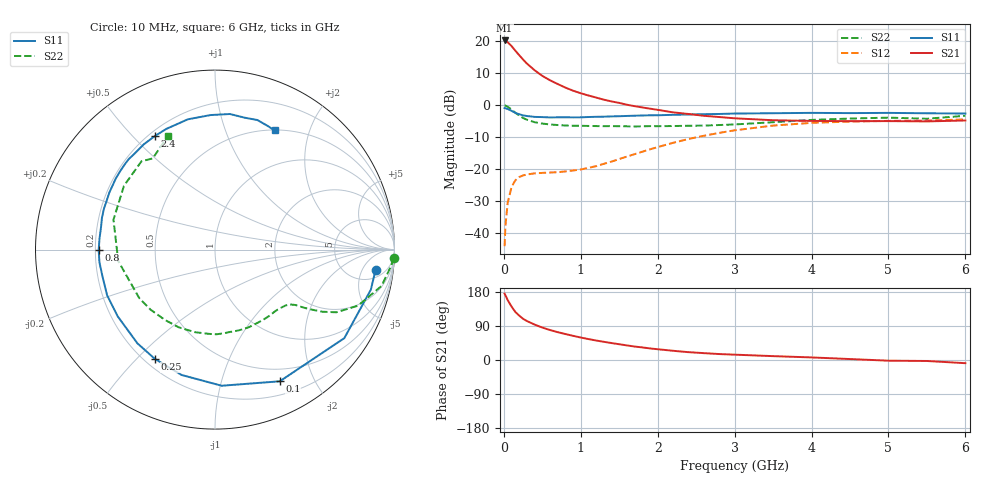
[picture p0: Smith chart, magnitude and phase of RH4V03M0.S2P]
! SIEMENS Small Signal Semiconductors
! BFR106
! Si NPN RF Bipolar Junction Transistor in SOT23
! VCE = 4 V  IC = 3 mA
! Common Emitter S-Parameters:  August  1996
# GHz  S  MA  R  50
!  f  S11  S21  S12  S22
! GHz  MAG  ANG  MAG  ANG  MAG  ANG  MAG  ANG
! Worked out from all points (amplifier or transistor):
!   36 points, 10 MHz to 6 GHz, reference 50 ohm
!   highest |S21| = 20.2 dB at 10 MHz (marker M1)
!   |S21| within 3 dB of that: start of sweep to 143.1 MHz
!   unconditionally stable (mu >= 1): 718.2 MHz to 1.879 GHz; 4.252 GHz to end of sweep
!   at 250 MHz: K = 0.39, MSG = 18.1 dB, |S12| = -21.9 dB
!   at 1.4 GHz: K = 1.20, MAG = 6.7 dB, |S12| = -17.6 dB
!   at 6 GHz: K = 1.02, MAG = -1.1 dB, |S12| = -4.4 dB
!   S11 on the Smith chart (normalised r, x): 10 MHz: 8, -10; 100 MHz: 0.35, -1.55; 250 MHz: 0.24, -0.57; 800 MHz: 0.21, -0.00; 2.4 GHz: 0.22, +0.58; 6 GHz: 0.51, +1.50
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0.01  0.902 -7.1  10.27 175.0  0.0063 87.1  0.9962 -2.7
0.02  0.8966 -14.4  10.24 171.1  0.0128 84.8  0.986 -5.2
0.05  0.8732 -34.4  9.603 158.0  0.03 72.7  0.9498 -12.3
0.1  0.8178 -63.8  8.413 141.1  0.0531 58.0  0.856 -21.4
0.15  0.7594 -87.2  7.1 126.6  0.0673 47.2  0.7614 -27.3
0.2  0.7229 -104.9  6.043 117.1  0.0756 41.3  0.6904 -30.1
0.25  0.695 -118.8  5.162 108.7  0.0802 36.7  0.6315 -31.9
0.3  0.678 -129.6  4.473 102.8  0.083 34.4  0.5938 -33.1
0.4  0.6574 -145.6  3.516 93.5  0.0863 31.6  0.5434 -34.6
0.5  0.6527 -157.1  2.873 85.6  0.0878 31.4  0.5171 -36.2
0.6  0.6445 -166.4  2.453 79.1  0.089 33.2  0.501 -38.5
0.8  0.6481 -179.8  1.885 68.5  0.0925 39.2  0.4825 -44.1
1.1  0.6545 164.2  1.419 55.2  0.1052 51.2  0.4749 -54.4
1.3  0.6625 155.5  1.221 48.0  0.1217 58.0  0.4712 -62.1
1.6  0.6802 144.3  1.018 38.5  0.1578 64.3  0.4685 -74.8
2.2  0.708 124.1  0.774 24.3  0.259 63.7  0.4735 -103.7
2.4  0.7162 117.8  0.73 20.7  0.2969 61.1  0.4778 -115.0
3.5  0.75 91.9  0.583 10.2  0.4811 38.5  0.5429 -173.3
4.5  0.7533 77.3  0.564 2.5  0.5557 17.4  0.6194 145.0
5  0.7596 71.9  0.565 -1.8  0.5695 9.1  0.6402 129.8
5.5  0.7486 66.8  0.559 -2.6  0.5753 5.1  0.6153 124.3
6  0.7426 63.4  0.578 -8.4  0.6009 -2.9  0.6844 112.5
